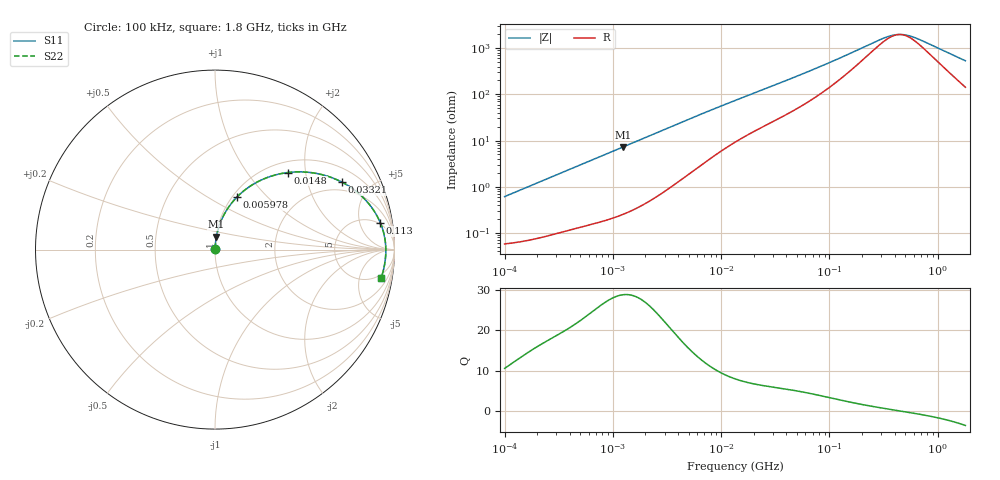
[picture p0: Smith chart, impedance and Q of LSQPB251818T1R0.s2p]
! LSQPB251818T1R0  S-PARAMETER MODEL  ( General Type )
! Model Generated by TAIYO YUDEN Corporation (http://www.ty-top.com)
! Version 2.0
! TAIYO YUDEN Control No. 100810NG19SB-FKC
! Copyright(c) 2009 TAIYO YUDEN CO.,LTD. All Rights Reserved.
! Product Description (link to TY-COMPAS)
! https://ds.yuden.co.jp/TYCOMPAS/or/detail?pn=LSQPB251818T1R0M&u=M
! Products Name : Inductors
! Characteristics :
!  Inductance : 1.0 uH , SRF(min) : 280 MHz , DC Resistance(max) : 0.065 Ohm
!  Rated Current : Saturation :2550 mA , Temp Rise : 1650 mA (40 degC)
!  Case Size : 2.5 x 1.8 / 0.098 x 0.071 [mm/inch] , Thickness : 1.8 / 0.071 [mm/inch]
!  (Conditions: Temperature = 25 degC , DC Bias Current/Voltage = 0A / 0V)
! External Node Assignments :
!  1  o---GGG---o  2
! GND o---------o GND
! Frequency Range : 0.1MHz  -  1800MHz  [ 402 STEP ]
# MHz S RI R 50
! Freq[MHz].  S11 Real  S11 Imag  S21 Real  S21 Imag  S12 Real  S12 Imag  S22 Real  S22 Imag
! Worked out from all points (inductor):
!   401 points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, 100 kHz to 1.8 GHz, reference 50 ohm
!   read as one part in series: L = 965 nH near 105 kHz
!   highest Q = 28.8 at 1.247 MHz (marker M1), where L = 930 nH
!   self-resonance near 443.9 MHz
!   S11 on the Smith chart (normalised r, x): 100 kHz: 1.00, +0.01; 5.978 MHz: 1.05, +0.68; 14.8 MHz: 1.21, +1.59; 33.21 MHz: 1.58, +3.31; 113 MHz: 5, +10; 1.8 GHz: 4, -10
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0.1  0.000613 0.00607  0.9994 -0.00607  0.9994 -0.00607  0.000613 0.00607
0.516129  0.00227 0.0304  0.9977 -0.0304  0.9977 -0.0304  0.00227 0.0304
1.246616  0.00776 0.0721  0.9922 -0.0721  0.9922 -0.0721  0.00776 0.0721
2.66389  0.0294 0.1491  0.9706 -0.1491  0.9706 -0.1491  0.0294 0.1491
4.140031  0.0652 0.2204  0.9348 -0.2204  0.9348 -0.2204  0.0652 0.2204
5.97828  0.1221 0.2925  0.8779 -0.2925  0.8779 -0.2925  0.1221 0.2925
8.84682  0.2208 0.3687  0.7792 -0.3687  0.7792 -0.3687  0.2208 0.3687
13.41641  0.3667 0.4231  0.6333 -0.4231  0.6333 -0.4231  0.3667 0.4231
14.79752  0.4049 0.4293  0.5951 -0.4293  0.5951 -0.4293  0.4049 0.4293
21.89777  0.56 0.4253  0.44 -0.4253  0.44 -0.4253  0.56 0.4253
33.20848  0.7075 0.3758  0.2925 -0.3758  0.2925 -0.3758  0.7075 0.3758
47.95365  0.8063 0.3081  0.1937 -0.3081  0.1937 -0.3081  0.8063 0.3081
69.24595  0.8726 0.2354  0.1274 -0.2354  0.1274 -0.2354  0.8726 0.2354
113.0207  0.921 0.1497  0.079 -0.1497  0.079 -0.1497  0.921 0.1497
286.6876  0.9496 0.0386  0.0504 -0.0386  0.0504 -0.0386  0.9496 0.0386
357.3983  0.9512 0.0187  0.0488 -0.0187  0.0488 -0.0187  0.9512 0.0187
445.5497  0.9519 -0.000327  0.0481 0.000327  0.0481 0.000327  0.9519 -0.000327
503.6016  0.9519 -0.0109  0.0481 0.0109  0.0481 0.0109  0.9519 -0.0109
569.2172  0.9516 -0.0216  0.0484 0.0216  0.0484 0.0216  0.9516 -0.0216
709.6131  0.9503 -0.0417  0.0497 0.0417  0.0497 0.0417  0.9503 -0.0417
1408.934  0.9367 -0.1209  0.0633 0.1209  0.0633 0.1209  0.9367 -0.1209
1800  0.925 -0.1591  0.075 0.1591  0.075 0.1591  0.925 -0.1591
